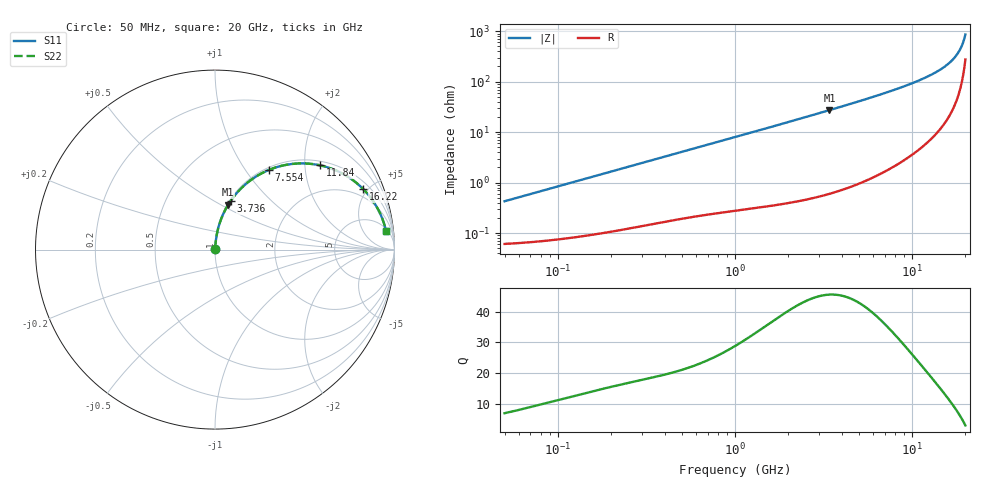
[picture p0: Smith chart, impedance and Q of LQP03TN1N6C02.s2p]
!Murata Part Number: LQP03TN1N6C02
!These Parameters are Measured in Series Mode Connection
!  o--[Z]--o
!Port1  Port2
!  o-------o
!Freq. Start=50[MHz] Stop=20[GHz], 401[Steps]
# Hz S RI R 50
!Freq.(Hz) S11(Real) S11(Imag) S21(Real) S21(Imag) S12(Real) S12(Imag) S22(Real) S22(Imag)
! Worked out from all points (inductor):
!   401 points, 50 MHz to 20 GHz, reference 50 ohm
!   read as one part in series: L = 1.35 nH near 51.52 MHz
!   highest Q = 45.5 at 3.415 GHz (marker M1), where L = 1.27 nH
!   S11 on the Smith chart (normalised r, x): 50 MHz: 1.00, +0.01; 3.736 GHz: 1.01, +0.60; 7.554 GHz: 1.04, +1.30; 11.84 GHz: 1.11, +2.39; 16.22 GHz: 1.42, +4.68; 20 GHz: 7, +16
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5e7  0.000628 0.00423  0.9994 -0.00423  0.9994 -0.00423  0.000628 0.00423
1.364002e8  0.000991 0.0114  0.999 -0.0114  0.999 -0.0114  0.000991 0.0114
3.721004e8  0.0025 0.0302  0.9975 -0.0302  0.9975 -0.0302  0.0025 0.0302
1e9  0.00899 0.0786  0.991 -0.0786  0.991 -0.0786  0.00899 0.0786
1.689197e9  0.021 0.1305  0.979 -0.1305  0.979 -0.1305  0.021 0.1305
2.728004e9  0.0492 0.2052  0.9508 -0.2052  0.9508 -0.2052  0.0492 0.2052
3.415248e9  0.0741 0.2513  0.9259 -0.2513  0.9259 -0.2513  0.0741 0.2513
3.736399e9  0.0874 0.2717  0.9126 -0.2717  0.9126 -0.2717  0.0874 0.2717
5.433528e9  0.172 0.3655  0.828 -0.3655  0.828 -0.3655  0.172 0.3655
6.406762e9  0.2292 0.4074  0.7708 -0.4074  0.7708 -0.4074  0.2292 0.4074
7.442007e9  0.2947 0.4416  0.7053 -0.4416  0.7053 -0.4416  0.2947 0.4416
7.554318e9  0.302 0.4446  0.698 -0.4446  0.698 -0.4446  0.302 0.4446
9.600142e9  0.4383 0.4782  0.5617 -0.4782  0.5617 -0.4782  0.4383 0.4782
1.183995e10  0.585 0.4696  0.415 -0.4696  0.415 -0.4696  0.585 0.4696
1.417136e10  0.7229 0.4166  0.2771 -0.4166  0.2771 -0.4166  0.7229 0.4166
1.527346e10  0.7806 0.3776  0.2194 -0.3776  0.2194 -0.3776  0.7806 0.3776
1.621653e10  0.8256 0.3375  0.1744 -0.3375  0.1744 -0.3375  0.8256 0.3375
1.721783e10  0.8684 0.2878  0.1316 -0.2878  0.1316 -0.2878  0.8684 0.2878
1.828096e10  0.9076 0.2261  0.0924 -0.2261  0.0924 -0.2261  0.9076 0.2261
1.88369e10  0.9252 0.1896  0.0748 -0.1896  0.0748 -0.1896  0.9252 0.1896
1.970266e10  0.9475 0.1255  0.0525 -0.1255  0.0525 -0.1255  0.9475 0.1255
2e10  0.9535 0.1011  0.0465 -0.1011  0.0465 -0.1011  0.9535 0.1011
